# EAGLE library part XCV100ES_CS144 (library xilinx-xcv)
xcv100es_cs144 edit this description Auto generated by make-symbol-device-package-bsdl.ulp Rev. 26 Source: xcv100es_cs144.bsd
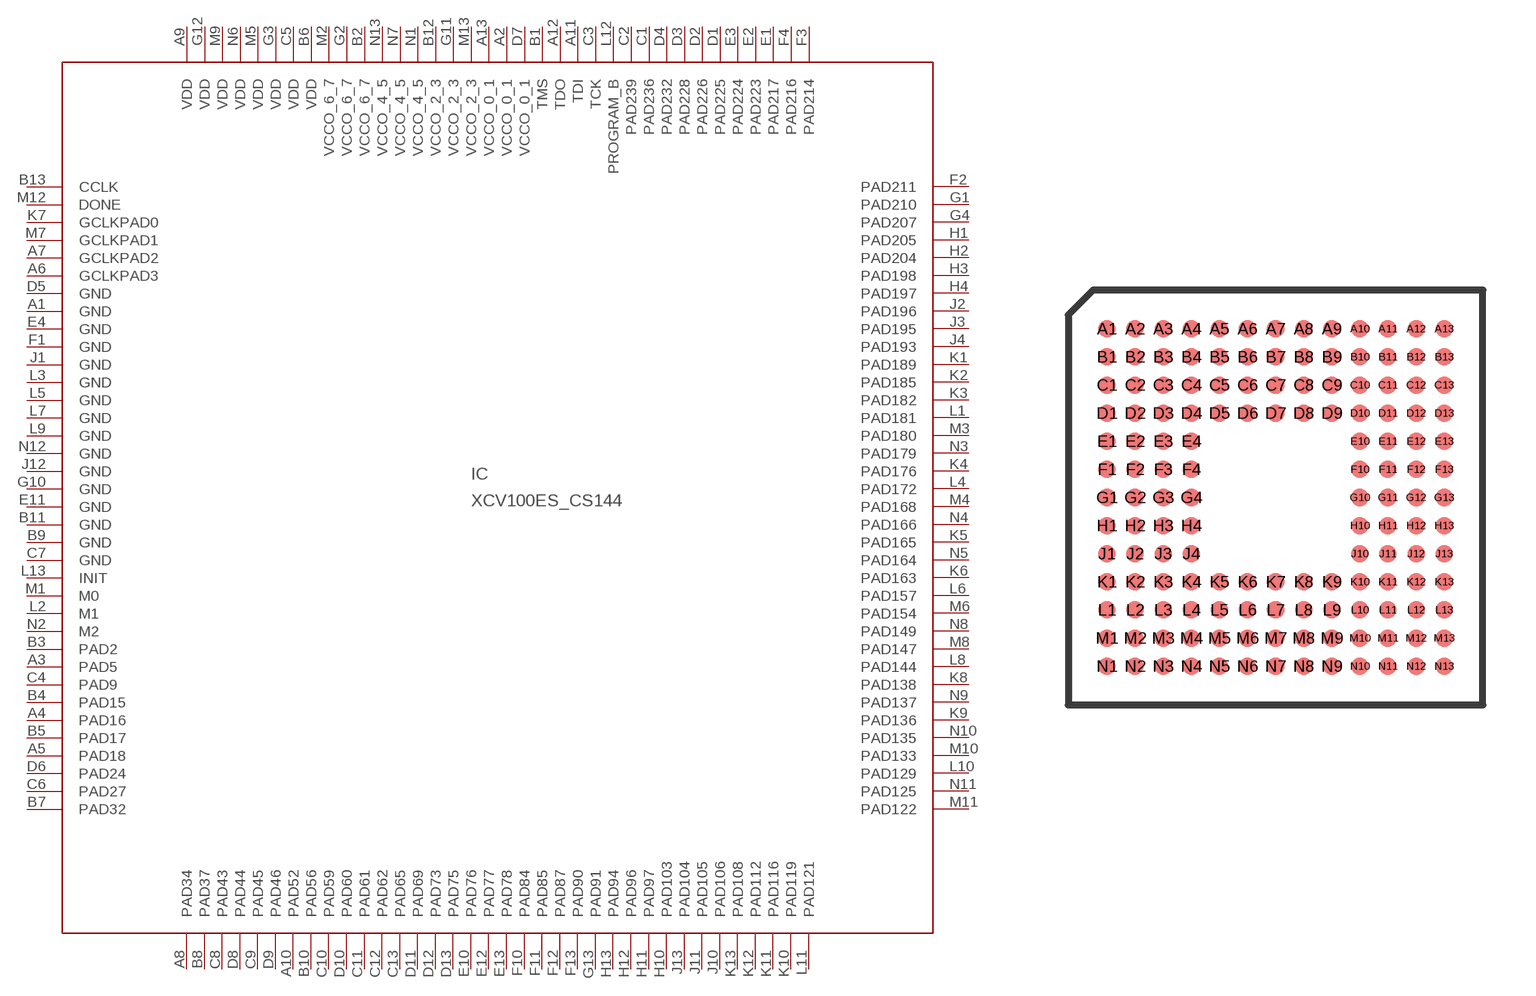
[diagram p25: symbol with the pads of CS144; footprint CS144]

Designator prefix IC

## XCV100ES_CS144 (OC_FARNELL: unknown; OC_NEWARK: unknown)  [CS144]
A1  GND  pwr
A2  VCCO_0_1  pwr
A3  PAD5
A4  PAD16
A5  PAD18
A6  GCLKPAD3  in
A7  GCLKPAD2  in
A8  PAD34
A9  VDD  pwr
A10  PAD52
A11  TDI  in
A12  TDO  out
A13  VCCO_0_1  pwr
B1  TMS  in
B2  VCCO_6_7  pwr
B3  PAD2
B4  PAD15
B5  PAD17
B6  VDD  pwr
B7  PAD32
B8  PAD37
B9  GND  pwr
B10  PAD56
B11  GND  pwr
B12  VCCO_2_3  pwr
B13  CCLK
C1  PAD236
C2  PAD239
C3  TCK  in
C4  PAD9
C5  VDD  pwr
C6  PAD27
C7  GND  pwr
C8  PAD43
C9  PAD45
C10  PAD59
C11  PAD61
C12  PAD62
C13  PAD65
D1  PAD225
D2  PAD226
D3  PAD228
D4  PAD232
D5  GND  pwr
D6  PAD24
D7  VCCO_0_1  pwr
D8  PAD44
D9  PAD46
D10  PAD60
D11  PAD69
D12  PAD73
D13  PAD75
E1  PAD217
E2  PAD223
E3  PAD224
E4  GND  pwr
E10  PAD76
E11  GND  pwr
E12  PAD77
E13  PAD78
F1  GND  pwr
F2  PAD211
F3  PAD214
F4  PAD216
F10  PAD84
F11  PAD85
F12  PAD87
F13  PAD90
G1  PAD210
G2  VCCO_6_7  pwr
G3  VDD  pwr
G4  PAD207
G10  GND  pwr
G11  VCCO_2_3  pwr
G12  VDD  pwr
G13  PAD91
H1  PAD205
H2  PAD204
H3  PAD198
H4  PAD197
H10  PAD103
H11  PAD97
H12  PAD96
H13  PAD94
J1  GND  pwr
J2  PAD196
J3  PAD195
J4  PAD193
J10  PAD106
J11  PAD105
J12  GND  pwr
J13  PAD104
K1  PAD189
K2  PAD185
K3  PAD182
K4  PAD176
K5  PAD165
K6  PAD163
K7  GCLKPAD0  in
K8  PAD138
K9  PAD136
K10  PAD119
K11  PAD116
K12  PAD112
K13  PAD108
L1  PAD181
L2  M1  in
L3  GND  pwr
L4  PAD172
L5  GND  pwr
L6  PAD157
L7  GND  pwr
L8  PAD144
L9  GND  pwr
L10  PAD129
L11  PAD121
L12  PROGRAM_B  in
L13  INIT
M1  M0  in
M2  VCCO_6_7  pwr
M3  PAD180
M4  PAD168
M5  VDD  pwr
M6  PAD154
M7  GCLKPAD1  in
M8  PAD147
M9  VDD  pwr
M10  PAD133
M11  PAD122
M12  DONE
M13  VCCO_2_3  pwr
N1  VCCO_4_5  pwr
N2  M2  in
N3  PAD179
N4  PAD166
N5  PAD164
N6  VDD  pwr
N7  VCCO_4_5  pwr
N8  PAD149
N9  PAD137
N10  PAD135
N11  PAD125
N12  GND  pwr
N13  VCCO_4_5  pwr

## Footprint CS144 (pad centres in mm)
xcv100e_cs144 edit this description Auto generated by make-symbol-device-package-bsdl.ulp Rev. 26 Source: xcv100e_cs144.bsd
smd 0.5 x 0.5: A1 -4.8,4.8; A2 -4,4.8; A3 -3.2,4.8; A4 -2.4,4.8; A5 -1.6,4.8; A6 -0.8,4.8; A7 0,4.8; A8 0.8,4.8; A9 1.6,4.8; A10 2.4,4.8; A11 3.2,4.8; A12 4,4.8; A13 4.8,4.8; B1 -4.8,4; B2 -4,4; B3 -3.2,4; B4 -2.4,4; B5 -1.6,4; B6 -0.8,4; B7 0,4; B8 0.8,4; B9 1.6,4; B10 2.4,4; B11 3.2,4; B12 4,4; B13 4.8,4; C1 -4.8,3.2; C2 -4,3.2; C3 -3.2,3.2; C4 -2.4,3.2; C5 -1.6,3.2; C6 -0.8,3.2; C7 0,3.2; C8 0.8,3.2; C9 1.6,3.2; C10 2.4,3.2; C11 3.2,3.2; C12 4,3.2; C13 4.8,3.2; D1 -4.8,2.4; D2 -4,2.4; D3 -3.2,2.4; D4 -2.4,2.4; D5 -1.6,2.4; D6 -0.8,2.4; D7 0,2.4; D8 0.8,2.4; D9 1.6,2.4; D10 2.4,2.4; D11 3.2,2.4; D12 4,2.4; D13 4.8,2.4; E1 -4.8,1.6; E2 -4,1.6; E3 -3.2,1.6; E4 -2.4,1.6; E10 2.4,1.6; E11 3.2,1.6; E12 4,1.6; E13 4.8,1.6; F1 -4.8,0.8; F2 -4,0.8; F3 -3.2,0.8; F4 -2.4,0.8; F10 2.4,0.8; F11 3.2,0.8; F12 4,0.8; F13 4.8,0.8; G1 -4.8,0; G2 -4,0; G3 -3.2,0; G4 -2.4,0; G10 2.4,0; G11 3.2,0; G12 4,0; G13 4.8,0; H1 -4.8,-0.8; H2 -4,-0.8; H3 -3.2,-0.8; H4 -2.4,-0.8; H10 2.4,-0.8; H11 3.2,-0.8; H12 4,-0.8; H13 4.8,-0.8; J1 -4.8,-1.6; J2 -4,-1.6; J3 -3.2,-1.6; J4 -2.4,-1.6; J10 2.4,-1.6; J11 3.2,-1.6; J12 4,-1.6; J13 4.8,-1.6; K1 -4.8,-2.4; K2 -4,-2.4; K3 -3.2,-2.4; K4 -2.4,-2.4; K5 -1.6,-2.4; K6 -0.8,-2.4; K7 0,-2.4; K8 0.8,-2.4; K9 1.6,-2.4; K10 2.4,-2.4; K11 3.2,-2.4; K12 4,-2.4; K13 4.8,-2.4; L1 -4.8,-3.2; L2 -4,-3.2; L3 -3.2,-3.2; L4 -2.4,-3.2; L5 -1.6,-3.2; L6 -0.8,-3.2; L7 0,-3.2; L8 0.8,-3.2; L9 1.6,-3.2; L10 2.4,-3.2; L11 3.2,-3.2; L12 4,-3.2; L13 4.8,-3.2; M1 -4.8,-4; M2 -4,-4; M3 -3.2,-4; M4 -2.4,-4; M5 -1.6,-4; M6 -0.8,-4; M7 0,-4; M8 0.8,-4; M9 1.6,-4; M10 2.4,-4; M11 3.2,-4; M12 4,-4; M13 4.8,-4; N1 -4.8,-4.8; N2 -4,-4.8; N3 -3.2,-4.8; N4 -2.4,-4.8; N5 -1.6,-4.8; N6 -0.8,-4.8; N7 0,-4.8; N8 0.8,-4.8; N9 1.6,-4.8; N10 2.4,-4.8; N11 3.2,-4.8; N12 4,-4.8; N13 4.8,-4.8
